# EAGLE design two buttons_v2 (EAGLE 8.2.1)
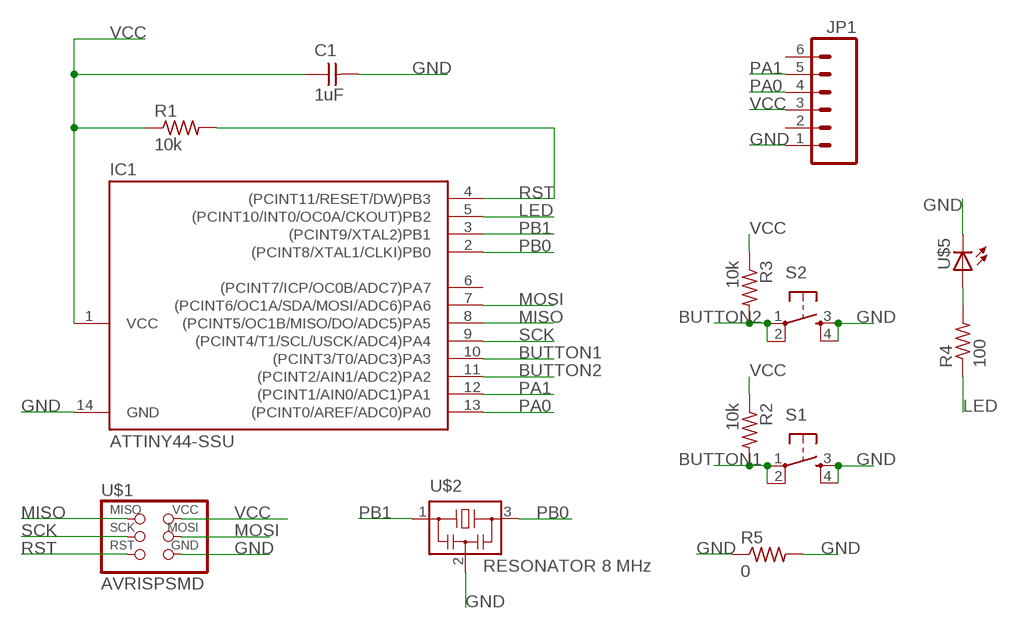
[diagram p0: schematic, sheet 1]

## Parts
C1  1uF  UNPOLARIZED_CAPACITOR1206  [1206]
IC1  ATTINY44-SSU  [SOIC14]
JP1  M06SMD  [1X06-SMD]
R1  10k  RESISTOR1206  [1206]
R2  10k  RESISTOR1206  [1206]
R3  10k  RESISTOR1206  [1206]
R4  100  RESISTOR1206  [1206]
R5  0  RESISTOR1206  [1206]
S1  6MM_SWITCH6MM_SWITCH  [6MM_SWITCH]
S2  6MM_SWITCH6MM_SWITCH  [6MM_SWITCH]
U$1  AVRISPSMD  [2X03SMD]
U$2  RESONATOR 8 MHz  RESONATOR  [EFOBM]
U$5  LED1206  [1206]

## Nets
BUTTON1: IC1.10((PCINT3/T0/ADC3)PA3) R2.2 S1.1(P) S1.2(P1)
BUTTON2: IC1.11((PCINT2/AIN1/ADC2)PA2) R3.2 S2.1(P) S2.2(P1)
GND: C1.2 IC1.14(GND) JP1.1 R5.1 R5.2 S1.3(S) S1.4(S1) S2.3(S) S2.4(S1) U$1.6(GND) U$2.2 U$5.2(C)
LED: IC1.5((PCINT10/INT0/OC0A/CKOUT)PB2) R4.1
MISO: IC1.8((PCINT5/OC1B/MISO/DO/ADC5)PA5) U$1.1(MISO)
MOSI: IC1.7((PCINT6/OC1A/SDA/MOSI/ADC6)PA6) U$1.4(MOSI)
N$1: R4.2 U$5.1(A)
PA0: IC1.13((PCINT0/AREF/ADC0)PA0) JP1.4
PA1: IC1.12((PCINT1/AIN0/ADC1)PA1) JP1.5
PB0: IC1.2((PCINT8/XTAL1/CLKI)PB0) U$2.3
PB1: IC1.3((PCINT9/XTAL2)PB1) U$2.1
RST: IC1.4((PCINT11/RESET/DW)PB3) R1.2 U$1.5(RST)
SCK: IC1.9((PCINT4/T1/SCL/USCK/ADC4)PA4) U$1.3(SCK)
VCC: C1.1 IC1.1(VCC) JP1.3 R1.1 R2.1 R3.1 U$1.2(VCC)
Unconnected: IC1.6((PCINT7/ICP/OC0B/ADC7)PA7) JP1.2 JP1.6

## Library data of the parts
C1 = 01_FAB_Hello:UNPOLARIZED_CAPACITOR: unpolarized_capacitor
IC1 = 01_FAB_Hello:ATTINY44
JP1 = SparkFun:M06: Header 6 Standard 6-pin 0.1" header. Use with straight break away headers (SKU : PRT-00116), right angle break away headers (PRT-00553), swiss pins (PRT-00743), machine pins (PRT-00117), and female headers (PRT-00115). Molex polarized connector foot print use with SKU : PRT-08094 with associated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
R1 = 01_FAB_Hello:RESISTOR
R2-R5 = 01_ng:RESISTOR
S1 S2 = 01_fab:6MM_SWITCH: OMRON SWITCH
U$1 = 01_FAB_Hello:AVRISP
U$2 = 01_fab:RESONATOR
U$5 = 01_ng:LED

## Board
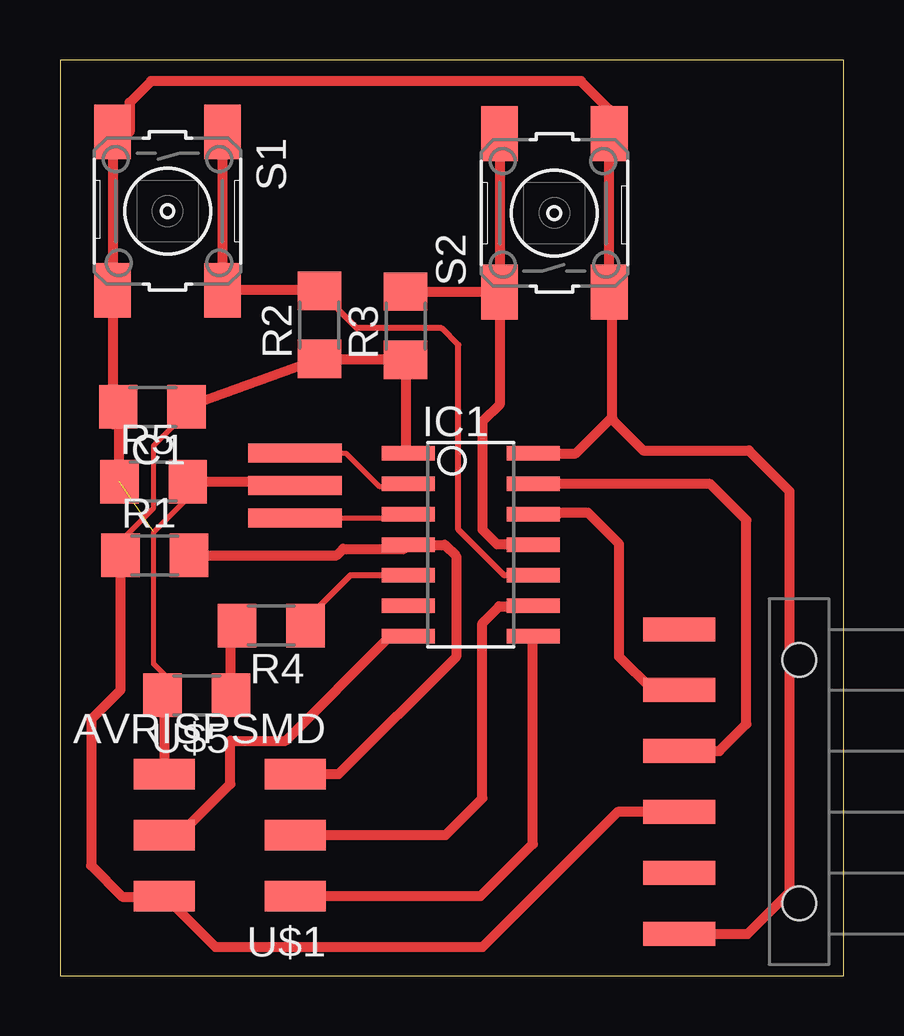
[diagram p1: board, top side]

Size 32.65 x 38.18 mm. Coordinates in mm from the lower left corner, seen from the top.
Outline: 0,0 32.65,0 32.65,38.18 0,38.18 0,0
Copper layers (1*16): Top 0.035mm / dielectric 1.5mm / Bottom 0.035mm
Design rules "default": minimum track width 10mil, minimum drill 24mil, track to track 8mil, track to pad 8mil, pad to pad 8mil, via to via 8mil, smd to smd 8mil, copper to edge 40mil, drill to drill 8mil, minimum pad ring 10mil, minimum via ring 8mil, stop-mask expansion 4mil, vias tented up to drill 0mil, thermal gap 10mil

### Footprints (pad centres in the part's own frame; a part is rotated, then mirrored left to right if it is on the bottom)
1206 = smd 1.6 x 1.803: 1 -1.422,0; 2 1.422,0
SOIC14 = smd 0.61 x 2.21: 1 -3.81,-2.603; 2 -2.54,-2.603; 3 -1.27,-2.603; 4 0,-2.603; 5 1.27,-2.603; 6 2.54,-2.603; 7 3.81,-2.603; 8 3.81,2.603; 9 2.54,2.603; 10 1.27,2.603; 11 0,2.603; 12 -1.27,2.603; 13 -2.54,2.603; 14 -3.81,2.603
1X06-SMD = smd 1 x 3: 1 -6.35,5; 2 -3.81,5; 3 -1.27,5; 4 1.27,5; 5 3.81,5; 6 6.35,5 | hole 1.4: -5.08,0; 5.08,0
6MM_SWITCH = smd 2.286 x 1.524: 1 -3.302,2.286; 2 3.302,2.286; 3 -3.302,-2.286; 4 3.302,-2.286
2X03SMD = smd 2.54 x 1.27: 1 -2.54,2.54; 2 2.92,2.54; 3 -2.54,0; 4 2.92,0; 5 -2.54,-2.54; 6 2.92,-2.54
EFOBM = smd 0.8 x 3.9: 1 -1.35,0; 2 0,0; 3 1.35,0

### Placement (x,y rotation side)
C1  3.85,23.72 180 top
IC1  17.11,17.97 270 top
JP1  30.8,8.1 90 top
R1  3.95,17.53 0 top
R2  10.81,27.14 90 top
R3  14.4,27.1 90 top
R4  8.8,14.6 180 top
R5  3.9,20.6 0 top
S1  4.48,31.88 270 top
S2  20.6,31.8 90 top
U$1  7.27,5.87 180 top
U$2  9.79,20.44 90 top
U$5  5.7,11.7 180 top

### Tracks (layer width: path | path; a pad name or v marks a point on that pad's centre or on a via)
BUTTON1
  Top 0.254: IC1.10 18.5,16.7 16.6,18.6 16.6,26.3 15.9,27 12.37,27 10.79,28.58
  Top 0.406: S1.1 S1.2 10.79,28.58 R2.2
BUTTON2
  Top 0.406: S2.2 S2.1 | S2.1 14.42,28.5 R3.2 | S2.1 18.31,23.81 17.6,23.1 17.6,18.6 18.2,18 19.68,18 IC1.11
GND  (1 unrouted)
  Top 0.152: 4.35,11.2 4.28,11.27 U$5.2 4.28,12.42 4.38,12.52
  Top 0.203: 4.38,12.52 3.9,13 3.9,18.5 5.4,20 5.4,20.52 R5.2
  Top 0.406: IC1.14 21.48,21.78 23,23.3 | 23,23.3 23,28.38 S2.3 S2.4 22.89,36.11 21.7,37.3 3.8,37.3 2.9,36.4 2.9,35.19 S1.3 S1.4 2.2,23 C1.2 R5.1 | 23,23.3 23,23.2 24.3,21.9 28.7,21.9 30.4,20.2 30.4,3.5 28.65,1.75 JP1.1 | 4.38,8.44 U$1.6 4.35,11.2 4.35,11.63 | R5.2 8,20.6 U$2.2
LED
  Top 0.254: R4.1 10.6,14.98 10.6,15.2 12.1,16.7 IC1.5
MISO
  Top 0.406: U$1.1 17.53,3.33 19.7,5.5 19.7,14.15 IC1.8
MOSI
  Top 0.406: U$1.4 4.97,5.87 7.1,8 7.1,9.8 9.4,9.8 13.7,14.1 14.45,14.1 IC1.7
N$1
  Top 0.406: U$5.1 7.12,14.34 R4.2
PA0
  Top 0.406: JP1.4 27.47,9.37 28.6,10.5 28.6,19 27.1,20.5 19.72,20.5 IC1.13
PA1
  Top 0.406: 20.7,19.2 19.75,19.2 IC1.12 19.77,19.3 22,19.3 23.3,18 23.3,13.3 24.69,11.91 JP1.5
PB0
  Top 0.203: U$2.3 11.91,21.79 13.3,20.4 14.4,20.4 IC1.2
PB1
  Top 0.203: U$2.1 14.36,19.09 IC1.3
RST
  Top 0.406: U$1.5 11.6,8.4 16.5,13.3 16.5,17.5 16.03,17.97 IC1.4 14.34,17.8 11.8,17.8 11.53,17.53 R1.2
SCK
  Top 0.406: U$1.3 16.07,5.87 17.6,7.4 17.6,14.7 18.3,15.4 19.68,15.4 IC1.9
VCC
  Top 0.203: C1.1 5.27,23.47 3.9,22.1 3.9,19.5 2.53,18.13 R1.1
  Top 0.406: IC1.1 14.4,21.89 R3.1 14.36,25.72 R2.1 C1.1 | JP1.3 23.23,6.83 17.6,1.2 6.48,1.2 U$1.2 4.32,3.3 2.6,3.3 1.3,4.6 1.3,10.7 2.53,11.93 R1.1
